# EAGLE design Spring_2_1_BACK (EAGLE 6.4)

## Sheet 1 of 2: Power
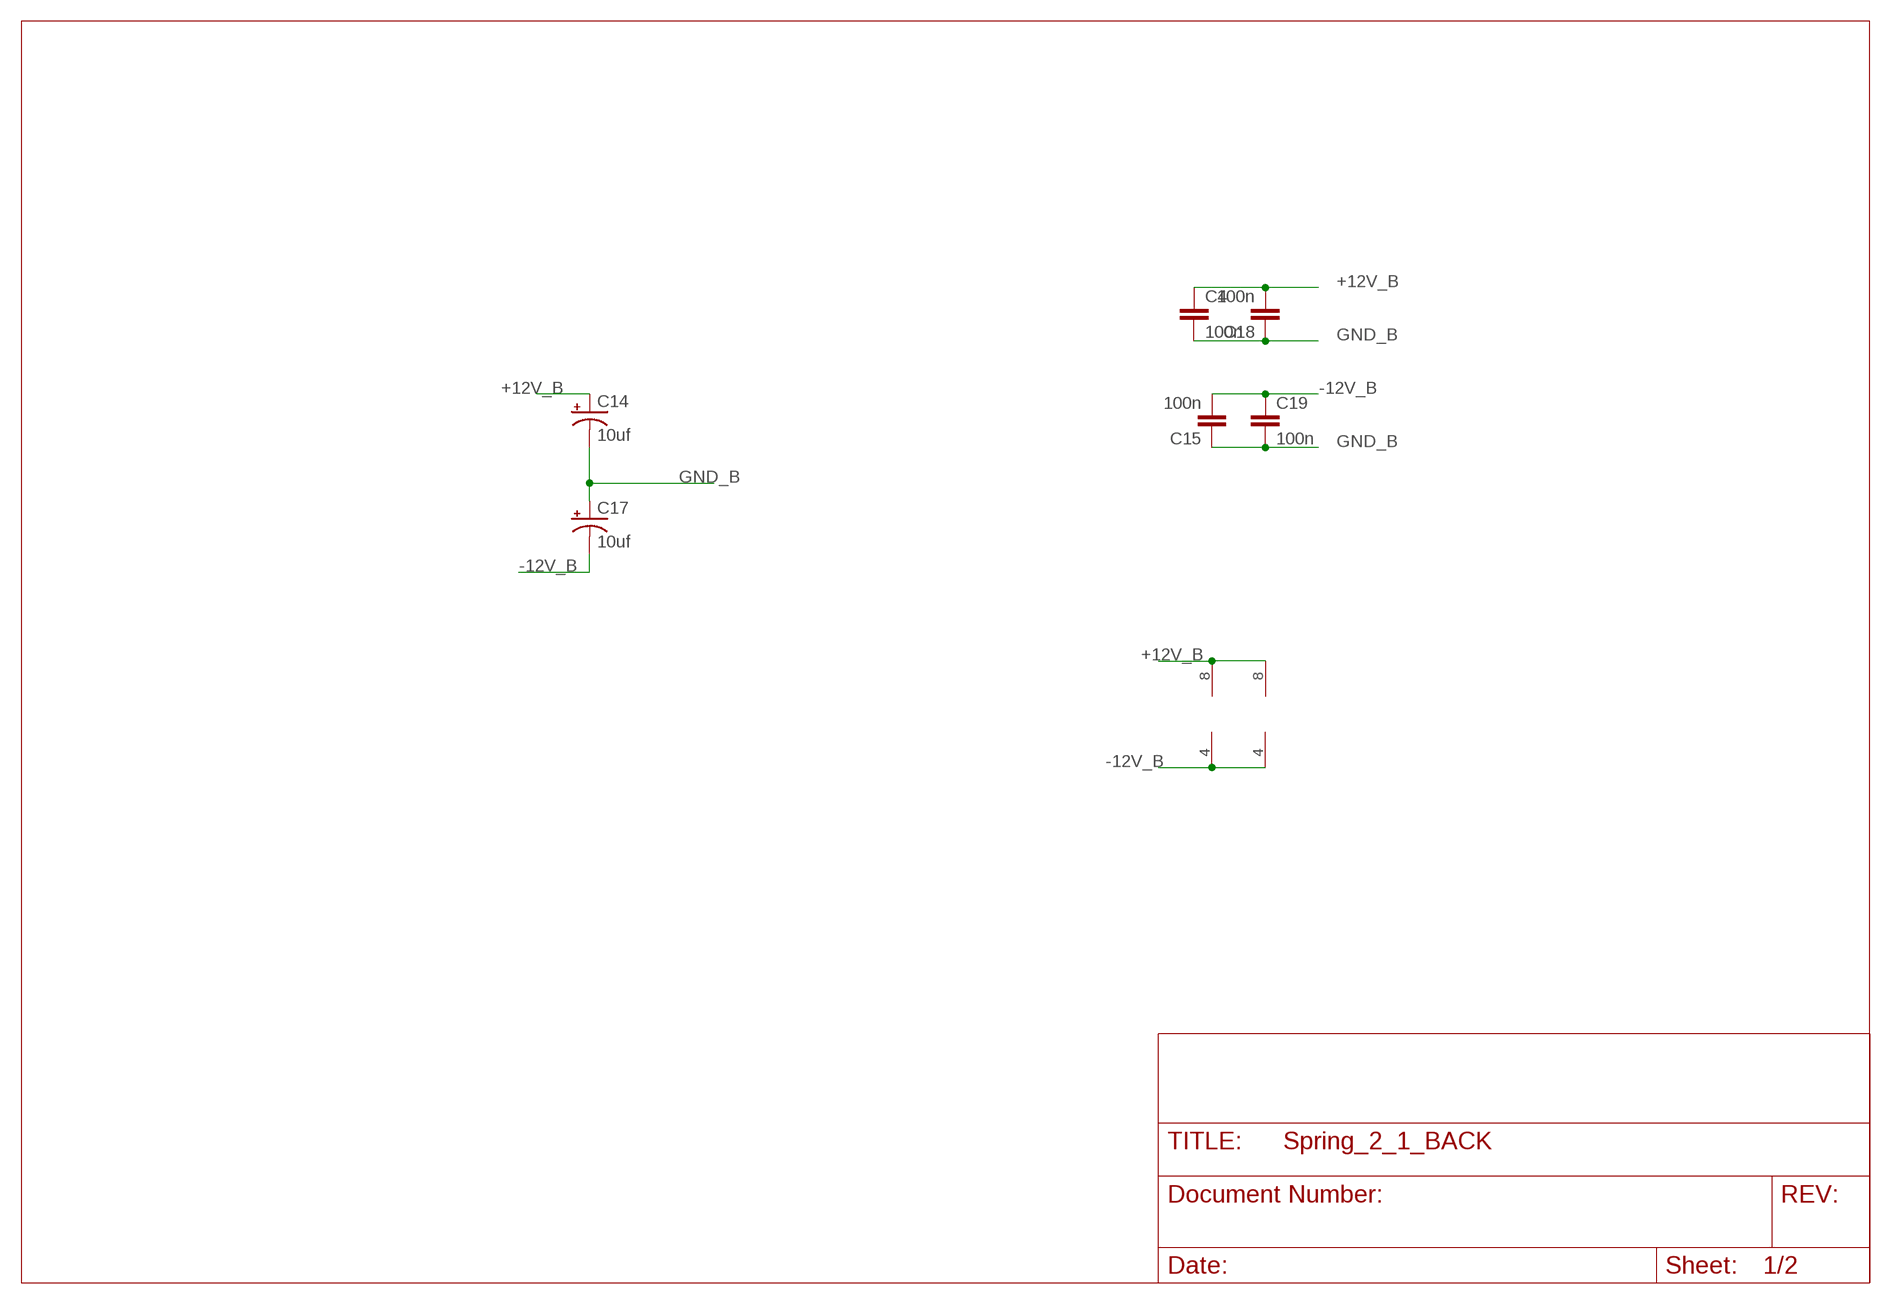
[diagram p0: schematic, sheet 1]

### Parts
BRICK  TL072  TL072P  [DIL08]
C4  100n  C-EU050-024X044  [C050-024X044]
C14  10uf  CAP_POLPTH2  [CPOL-RADIAL-10UF-25V]
C15  100n  C-EU050-024X044  [C050-024X044]
C17  10uf  CAP_POLPTH2  [CPOL-RADIAL-10UF-25V]
C18  100n  C-EU050-024X044  [C050-024X044]
C19  100n  C-EU050-024X044  [C050-024X044]
IC4_DRV_RCVR  TL072  TL072P  [DIL08]

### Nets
+12V_B [power]: BRICK.8(P:V+) C4.1 C14.1(+) C18.2 IC4_DRV_RCVR.8(P:V+) ; also sheet 2
-12V_B [power]: BRICK.4(P:V-) C15.2 C17.2(-) C19.1 IC4_DRV_RCVR.4(P:V-) ; also sheet 2
GND_B [ground]: C4.2 C14.2(-) C15.1 C17.1(+) C18.1 C19.2 ; also sheet 2

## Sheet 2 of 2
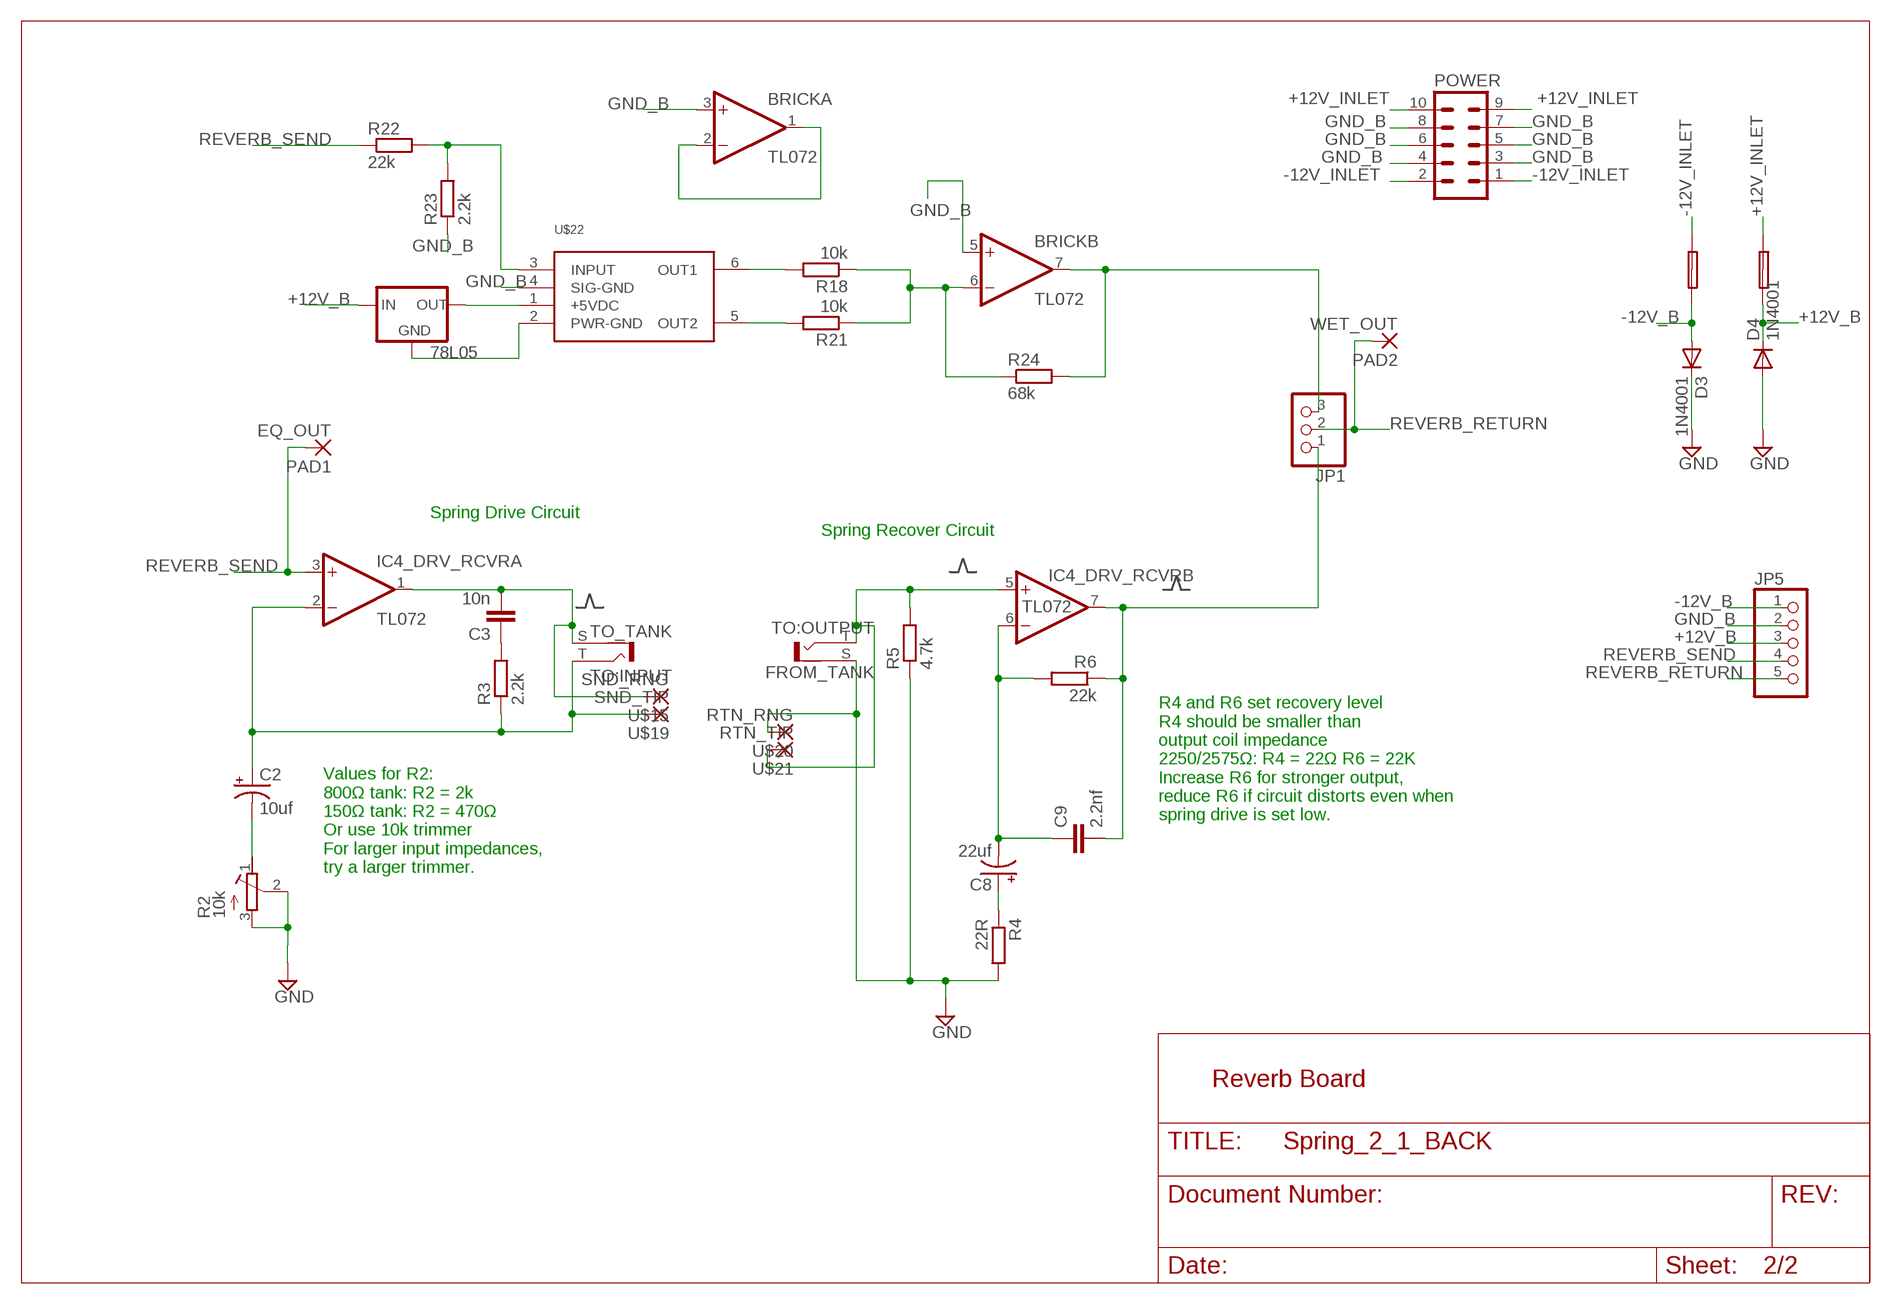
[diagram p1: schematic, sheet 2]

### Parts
0.1A_FUSE  FUSE  PTC_FUSEPOLY_FUSE  [C050H075X075]
0.1A_FUSE_2  FUSE  PTC_FUSEPOLY_FUSE  [C050H075X075]
78L05  V_REG_78XXTO-92  [TO-92]
C2  10uf  CAP_POLPTH2  [CPOL-RADIAL-10UF-25V]
C3  10n  C-EU050-024X044  [C050-024X044]
C8  22uf  CAP_POLPTH2  [CPOL-RADIAL-10UF-25V]
C9  2.2nf  C-EU050-024X044  [C050-024X044]
D3  1N4001  1N4004  [DO41-10]
D4  1N4001  1N4004  [DO41-10]
JP1  PINHD-1X3  [1X03]
JP5  PINHD-1X5  [1X05]
PAD1  EQ_OUT  LONG_PAD_1  [LONG_PAD_1]
PAD2  WET_OUT  LONG_PAD_1  [LONG_PAD_1]
POWER  10_PIN_HEADER  [MA05-2]
R2  10k  R-TRIMMT93YA  [RTRIMT93YA]
R3  2.2k  R-EU_STANDARD_RESISTOR  [0207/10]
R4  22R  R-EU_STANDARD_RESISTOR  [0207/10]
R5  4.7k  R-EU_STANDARD_RESISTOR  [0207/10]
R6  22k  R-EU_STANDARD_RESISTOR  [0207/10]
R18  10k  R-EU_STANDARD_RESISTOR  [0207/10]
R21  10k  R-EU_STANDARD_RESISTOR  [0207/10]
R22  22k  R-EU_STANDARD_RESISTOR  [0207/10]
R23  2.2k  R-EU_STANDARD_RESISTOR  [0207/10]
R24  68k  R-EU_STANDARD_RESISTOR  [0207/10]
TO:INPUT  TO_TANK  BTOR1  [BTOR1]
TO:OUTPUT  FROM_TANK  BTOR1  [BTOR1]
U$15  SND_RNG  LONG_PAD_1  [LONG_PAD_1]
U$19  SND_TIP  LONG_PAD_1  [LONG_PAD_1]
U$20  RTN_RNG  LONG_PAD_1  [LONG_PAD_1]
U$21  RTN_TIP  LONG_PAD_1  [LONG_PAD_1]
U$22  BTDR-2H  [BTDR-2H]

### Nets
+12V_B [power]: 0.1A_FUSE_2.1 78L05.3(IN) D4.C JP5.3 ; also sheet 1
+12V_INLET: 0.1A_FUSE_2.2 POWER.9 POWER.10
-12V_B [power]: 0.1A_FUSE.1 D3.A JP5.1 ; also sheet 1
-12V_INLET: 0.1A_FUSE.2 POWER.1 POWER.2
GND_B [ground]: BRICK.3(A:+IN) BRICK.5(B:+IN) D3.C D4.A JP5.2 POWER.3 POWER.4 POWER.5 POWER.6 POWER.7 POWER.8 R2.2(S) R2.3(E) R4.2 R5.1 R23.1 TO:OUTPUT.S U$20.P$1(P) U$22.4(SIG-GND) ; supply symbol labelled GND ; also sheet 1
N$1: C2.2(-) R2.1(A)
N$2: C3.1 R3.2
N$4: C3.2 IC4_DRV_RCVR.1(A:OUT) TO:INPUT.S U$15.P$1(P)
N$5: C2.1(+) IC4_DRV_RCVR.2(A:-IN) R3.1 TO:INPUT.T U$19.P$1(P)
N$7: IC4_DRV_RCVR.5(B:+IN) R5.2 TO:OUTPUT.T U$21.P$1(P)
N$8: C8.1(+) R4.1
N$9: C8.2(-) C9.1 IC4_DRV_RCVR.6(B:-IN) R6.2
N$19: 78L05.1(OUT) U$22.1(+5VDC)
N$27: R22.2 R23.2 U$22.3(INPUT)
N$28: R18.2 U$22.6(OUT1)
N$29: R21.2 U$22.5(OUT2)
N$30: BRICK.6(B:-IN) R18.1 R21.1 R24.1
N$32 [ground]: 78L05.2(GND) U$22.2(PWR-GND)
N$34: BRICK.1(A:OUT) BRICK.2(A:-IN)
N$38: BRICK.7(B:OUT) JP1.3 R24.2
N$39: C9.2 IC4_DRV_RCVR.7(B:OUT) JP1.1 R6.1
REVERB_RETURN: JP1.2 JP5.5 PAD2.P$1(P)
REVERB_SEND: IC4_DRV_RCVR.3(A:+IN) JP5.4 PAD1.P$1(P) R22.1
Unconnected: TO:INPUT.S@1 TO:INPUT.S@2 TO:INPUT.S@3 TO:OUTPUT.S@1 TO:OUTPUT.S@2 TO:OUTPUT.S@3

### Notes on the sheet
- Spring Drive Circuit
- Spring Recover Circuit
- Values for R2:
  800Ω tank: R2 = 2k
  150Ω tank: R2 = 470Ω
  Or use 10k trimmer
  For larger input impedances, 
  try a larger trimmer.
- R4 and R6 set recovery level 
  R4 should be smaller than 
  output coil impedance
  2250/2575Ω: R4 = 22Ω R6 = 22K 
  Increase R6 for stronger output, 
  reduce R6 if circuit distorts even when 
  spring drive is set low.
- Reverb Board

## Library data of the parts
0.1A_FUSE 0.1A_FUSE_2 = TomW:PTC_FUSE
78L05 = SparkFun-PowerIC:V_REG_78XX: Voltage Regulator Standard 7805 5V regulator. IGO (Input Ground Output). Spark Fun Electronics SKU : COM-00107
BRICK IC4_DRV_RCVR = TomW:TL072: OP AMP
C2 C8 C14 C17 = SparkFun-Passives:CAP_POL: Capacitor Polarized
C3 C4 C9 C15 C18 C19 = TomW:C-EU: CAPACITOR, European symbol
D3 D4 = diode:1N4004: DIODE
JP1 = pinhead:PINHD-1X3: PIN HEADER
JP5 = pinhead:PINHD-1X5: PIN HEADER
PAD1 PAD2 U$15 U$19-U$21 = TomW:LONG_PAD_1
POWER = TomW:10_PIN_HEADER: PIN HEADER; OC_FARNELL: unknown; OC_NEWARK: unknown
R2 = resistor:R-TRIMM: Trimm resistor
R3-R6 R18 R21-R24 = TomW:R-EU_: RESISTOR, European symbol
TO:INPUT TO:OUTPUT = con-lumberg:BTOR1: RCA connectors according to JEITA RC-5231 Cinch RCA-Einbaukupplung nach JEITA RC-5231, stehende Ausführung Source: http://www.lumberg.de/Produkte/PDFs/BTOR1.pdf; MPN: BTOR 1; OC_FARNELL: 1217030; OC_NEWARK: 96K7172
U$22 = Accutronics BTDR-2H:BTDR-2H: Accutronics BTDR-2H Information: http://www.accutronicsreverb.com/main/?skin=sub01_05_1.html

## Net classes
0 default: width 0.61 mm
1 power: width 0.914 mm
2 ground: width 0.914 mm

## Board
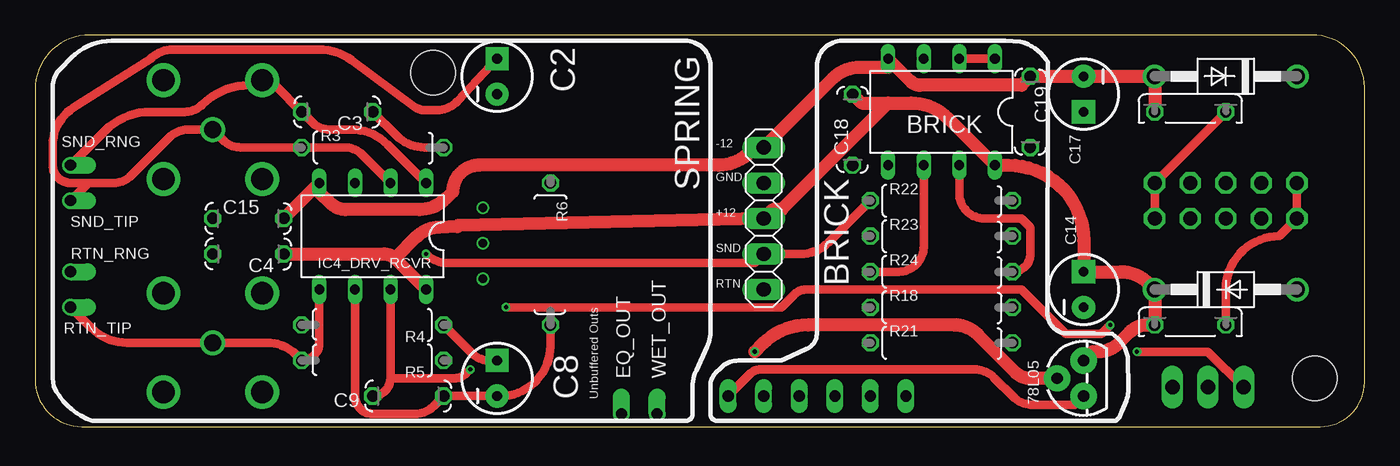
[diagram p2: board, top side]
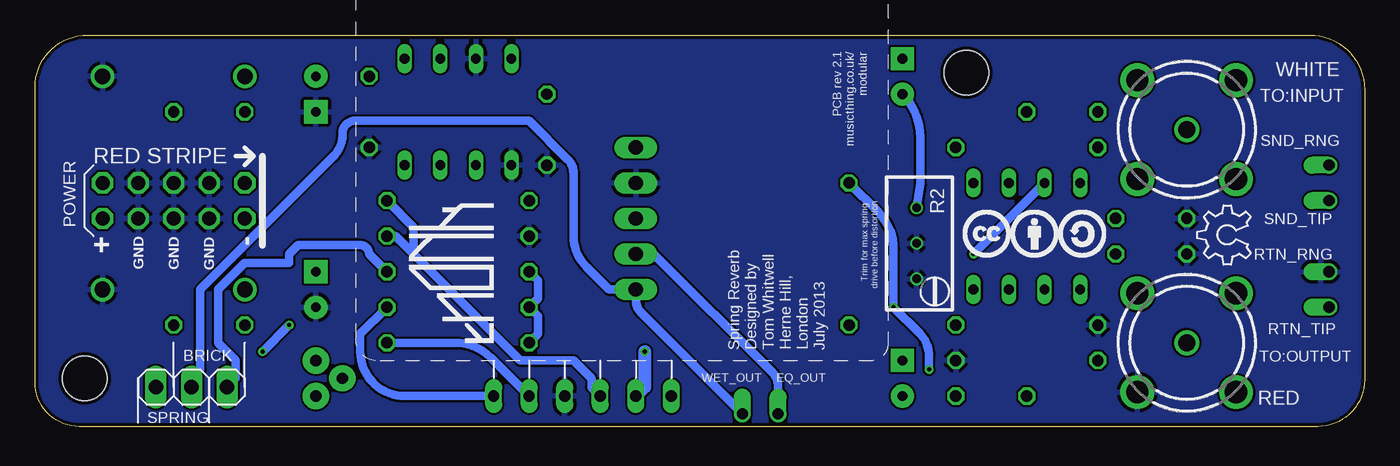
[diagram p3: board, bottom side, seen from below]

Size 95 x 28 mm. Coordinates in mm from the lower left corner, seen from the top.
Outline: 0,24.1 0,3.35 arc90 3.35,0 91.84,0 arc90 95,3.16 95,24.26 arc90 91.26,28 3.9,28 arc90 0,24.1
Copper layers (1*2*15*16): Top 0.035mm / dielectric 0.2mm / Route2 0.0175mm / dielectric 1.1mm / Route15 0.0175mm / dielectric 0.2mm / Bottom 0.035mm
Design rules "SeeedStudio_DRU_no_angle_20130527 *": minimum track width 6mil, minimum drill 12mil, track to track 6mil, track to pad 6mil, pad to pad 6mil, via to via 6mil, smd to smd 0mil, copper to edge 10mil, drill to drill 10mil, minimum pad ring 6mil, minimum via ring 6mil, stop-mask expansion 2mil, vias tented up to drill 25mil, thermal gap 10mil
Holes 3.2 mm at 28.45,25.29 91.44,3.45

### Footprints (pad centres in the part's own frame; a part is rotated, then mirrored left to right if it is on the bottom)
C050H075X075 = drill 0.813 octagon: 1 -2.54,0; 2 2.54,0
TO-92 = drill 0.813 pad 1.88: 1 -1.27,0; 2 0,1.905; 3 1.27,0
DIL08 = drill 0.7 long: 1 -3.81,-3.81; 2 -1.27,-3.81; 3 1.27,-3.81; 4 3.81,-3.81; 5 3.81,3.81; 6 1.27,3.81; 7 -1.27,3.81; 8 -3.81,3.81
CPOL-RADIAL-10UF-25V = drill 0.7 pad 1.651 square: 1 1.27,0 | drill 0.7 pad 1.651: 2 -1.27,0
C050-024X044 = drill 0.813 octagon: 1 -2.54,0; 2 2.54,0
DO41-10 = drill 1.118: A 5.08,0; C -5.08,0
1X03 = drill 1.016 long: 1 -2.54,0; 2 0,0; 3 2.54,0
1X05 = drill 1.016 long: 1 -5.08,0; 2 -2.54,0; 3 0,0; 4 2.54,0; 5 5.08,0
LONG_PAD_1 = drill 0.8 offset: P$1 0,0
MA05-2 = drill 1.016 octagon: 1 -5.08,-1.27; 2 -5.08,1.27; 3 -2.54,-1.27; 4 -2.54,1.27; 5 0,-1.27; 6 0,1.27; 7 2.54,-1.27; 8 2.54,1.27; 9 5.08,-1.27; 10 5.08,1.27
RTRIMT93YA = drill 0.61: 1 0,-2.54; 2 0,0; 3 0,2.54
0207/10 = drill 0.813 octagon: 1 -5.08,0; 2 5.08,0
BTOR1 = drill 1.6 pad 2.2: S -5,0; S@1 0,5; S@2 5,0; S@3 0,-5 | drill 1.2 pad 1.6: T 0,0
BTDR-2H = drill 0.8 long: 1 2.54,-17.78; 2 0,-17.78; 3 -2.54,-17.78; 4 -5.08,-17.78; 5 -7.62,-17.78; 6 -10.16,-17.78

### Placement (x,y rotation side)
0.1A_FUSE  82.55,22.5 0 top
0.1A_FUSE_2  82.55,7.26 0 top
78L05  74.93,3.45 90 top
BRICK  64.77,22.5 180 top
C2  33.02,25.04 90 top
C3  21.59,22.5 180 top
C4  15.24,12.34 180 top
C8  33.02,3.45 90 top
C9  26.67,2.18 180 top
C14  74.93,9.8 90 top
C15  15.24,14.88 0 top
C17  74.93,23.77 270 top
C18  58.42,21.23 90 top
C19  71.12,22.5 270 top
D3  85.09,25.04 180 top
D4  85.09,9.8 0 top
IC4_DRV_RCVR  24.13,13.61 180 top
JP1  83.82,2.81 0 bottom
JP5  52.07,14.88 270 top
PAD1  41.91,0.91 90 top
PAD2  44.45,0.91 90 top
POWER  85.09,16.15 180 bottom
R2  32,13.1 180 bottom
R3  24.13,19.96 0 top
R4  24.13,7.26 180 top
R5  24.13,4.72 180 top
R6  36.83,12.34 270 top
R18  64.77,8.53 0 top
R21  64.77,5.99 0 top
R22  64.77,16.15 0 top
R23  64.77,13.61 0 top
R24  64.77,11.07 0 top
TO:INPUT  12.7,21.23 315 bottom
TO:OUTPUT  12.7,5.99 45 bottom
U$1  [CC_1CM_SCREENPRINT]  28.7,12.09 0 bottom
U$2  [MTM_1CM_KEEPOUT]  40.89,15.39 90 bottom
U$3  [OSHW_6X150_NOTEXT]  8.13,11.58 90 bottom
U$4  [THONK_1CM_SCREENPRINT]  62.23,5.99 90 bottom
U$15  2.54,18.69 0 top
U$19  2.54,16.15 0 top
U$20  2.54,11.07 0 top
U$21  2.54,8.53 0 top
U$22  52.07,19.96 0 bottom

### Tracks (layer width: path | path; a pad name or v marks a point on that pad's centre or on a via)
+12V_B
  Top 0.914: 60.96,23.14 62.6,23.14 arc-45 65.22,22.05 BRICK.8 69.54,18.69 arc-90 74.93,13.3 C14.1 77.56,11.07 arc-45 79.57,10.24 D4.C 0.1A_FUSE_2.1 79.48,7.26 arc45 78.21,6.73 77.42,5.94 arc-45 76,5.35 75.56,5.35 78L05.3 | 60.96,23.14 59.05,23.14 C18.2 | 60.96,23.14 53.34,15.52 52.7,15.52 JP5.3 30.24,14.38 arc45 30.19,14.3 28.89,14.25 arc45 27.27,13.57 25.72,12.02 | C4.1 24.95,12.34 arc-45 25.72,12.02 | 25.72,12.02 IC4_DRV_RCVR.8
+12V_INLET
  Top 0.61: POWER.9 POWER.10 88.9,13.61 arc90 85.09,9.8 0.1A_FUSE_2.2
-12V_B
  Top 0.914: 0.1A_FUSE.1 D3.A C17.2 C19.1 70.48,24.41 63.24,24.41 arc-45 62.6,24.67 BRICK.4 60.96,25.68 58.9,25.68 arc45 57,24.89 JP5.1 51.44,19.96 51.09,19.62 arc-45 48.85,18.69 31.75,18.69 arc90 29.84,16.79 29.36,16.3 arc-45 27.46,15.52 22.18,15.52 arc-45 21.17,15.93 20.32,16.79 IC4_DRV_RCVR.4 C15.2
-12V_INLET
  Top 0.61: 0.1A_FUSE.2 POWER.1 POWER.2
GND_B
  pour Bottom: -2.54,-4.17 97.79,-1.63 97.79,31.39 -3.81,31.39
N$1
  Bottom 0.61: C2.2 arc45 31.75,20.7 31.75,17.42 R2.1
N$2
  Top 0.61: R3.2 27.85,19.96 arc-45 25.84,20.79 C3.1
N$4
  Top 0.61: IC4_DRV_RCVR.1 25.18,20.18 arc45 22.64,21.23 21.06,21.23 arc-45 19.79,21.76 C3.2 17.14,24.41 16.51,24.41 TO:INPUT.S 15.88,24.41 15.29,24.41 arc45 11.96,23.03 arc-45 10.69,22.5 8.25,22.5 arc45 5.01,21.16 U$15.P$1
N$5
  Top 0.61: IC4_DRV_RCVR.2 23.39,19.43 arc45 22.12,19.96 R3.1 14.71,19.96 arc-45 13.44,20.49 TO:INPUT.T 10.9,21.23 arc45 9.63,20.7 6.88,17.95 arc-45 5.61,17.42 3.81,17.42 | 3.81,17.42 U$19.P$1 | C2.1 30.19,23.27 arc-47 28.72,22.63 27.84,22.63 arc-36 27.1,22.87 22.61,26.19 arc36 20.32,26.95 9.84,26.95 arc45 8.22,26.27 2.74,22.8 arc58 1.27,20.12 1.27,18.69 arc90 2.54,17.42 3.81,17.42
  Bottom 0.61: IC4_DRV_RCVR.2 25.4,18.05
N$7
  Top 0.61: IC4_DRV_RCVR.5 20.32,5.99 arc-90 R5.2 18.61,5.16 arc45 16.6,5.99 TO:OUTPUT.T 6.57,5.99 arc-45 4.03,7.04 U$21.P$1
N$8
  Top 0.61: C8.1 32.49,4.72 arc-45 31.22,5.25 R4.1
N$9
  Top 0.61: IC4_DRV_RCVR.6 22.86,2.18 arc90 24.13,0.91 27.2,0.91 arc45 28.47,1.44 C9.1 C8.2 33.24,2.18 arc90 36.83,5.77 R6.2
N$19
  Top 0.61: U$22.1 51.17,3.82 arc-45 51.81,4.08 67.11,4.08 arc-45 68.53,3.5 69.9,2.13 arc45 71.32,1.54 74.3,1.54 78L05.1
N$27
  Bottom 0.61: U$22.3 55.24,2.81 55.24,3.45 56.52,4.72 60.33,4.72 67.94,12.34 | 67.94,12.34 69.22,13.61 R23.2 | R22.2 67.94,14.25 67.94,12.34
N$28
  Bottom 0.61: U$22.6 68.58,2.18 arc90 71.75,5.35 71.75,6.62 R18.2
N$29
  Bottom 0.61: R21.2 64.99,5.99 arc45 62.45,4.94 U$22.5
N$30
  Top 0.61: R24.1 61.7,11.07 arc90 63.5,12.87 BRICK.6
  Bottom 0.61: R21.1 59.05,6.62 59.05,7.9 R18.1 59.05,9.17 59.05,10.44 R24.1
N$32  (via drill 0.3)
  Top 0.914: v51.44,5.35 52,5.92 arc-45 55.24,7.26 65.73,7.26 arc-45 67.35,6.59 70.07,3.87 arc45 71.07,3.45 78L05.2
  Bottom 0.914: U$22.2 51.44,2.81 v51.44,5.35
N$34
  Top 0.61: BRICK.1 BRICK.2
N$38
  Top 0.61: BRICK.7 66.04,16.68 arc90 67.84,14.88 70.48,14.88 71.12,14.25 71.12,12.34 arc-90 R24.2
  Bottom 0.61: JP1.3 80.64,3.45 80.64,4.72 81.92,5.99 81.92,9.8 80.01,11.71 76.83,11.71 76.83,12.34 76.2,12.98 71.75,12.98 arc90 71.12,12.34 R24.2
N$39  (via drill 0.3)
  Top 0.61: C9.2 arc90 25.4,3.45 | 25.4,3.45 IC4_DRV_RCVR.7 | 25.4,3.45 29.95,3.45 arc45 30.85,3.82 v31.11,4.08 | JP1.1 83.82,5.35 v78.74,5.35 | v76.83,7.26 76.2,6.62 73.66,6.62 70.48,9.8 55.14,9.8 arc45 54.24,9.43 53.34,8.53 v33.66,8.53
  Bottom 0.61: R6.1 34.74,15.33 arc45 33.66,12.71 v33.66,8.53 31.79,6.66 arc45 31.11,5.04 v31.11,4.08 | v76.83,7.26 v78.74,5.35
REVERB_RETURN
  Bottom 0.61: JP1.2 83.82,3.45 83.19,4.08 83.19,9.8 73.7,19.29 arc-45 73.03,20.91 73.03,20.97 arc90 72.13,21.87 59.69,21.87 56.93,19.11 arc45 56.52,18.1 56.52,13.66 arc-45 55.59,11.41 53.98,9.8 JP5.5 52.07,9.06 arc-45 51.7,8.16 PAD2.P$1
REVERB_SEND  (via drill 0.3)
  Top 0.61: R22.1 56.71,13.17 arc-45 54.7,12.34 JP5.4 51.44,11.71 29.41,11.71 arc-45 27.99,12.29 v27.94,12.34
  Bottom 0.61: v27.94,12.34 IC4_DRV_RCVR.3 | PAD1.P$1 41.91,2.92 arc-45 42.28,3.82 50.8,12.34 JP5.4

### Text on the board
tPlace: -12 | GND | SPRING | +12 | SND | RTN | BRICK | Unbuffered Outs
bPlace: PCB rev 2.1 / musicthing.co.uk/ / modular | WHITE | Trim for max spring / drive before distortion | Spring Reverb / Designed by / Tom Whitwell / Herne Hill, / London / July 2013 | BRICK | RED | SPRING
